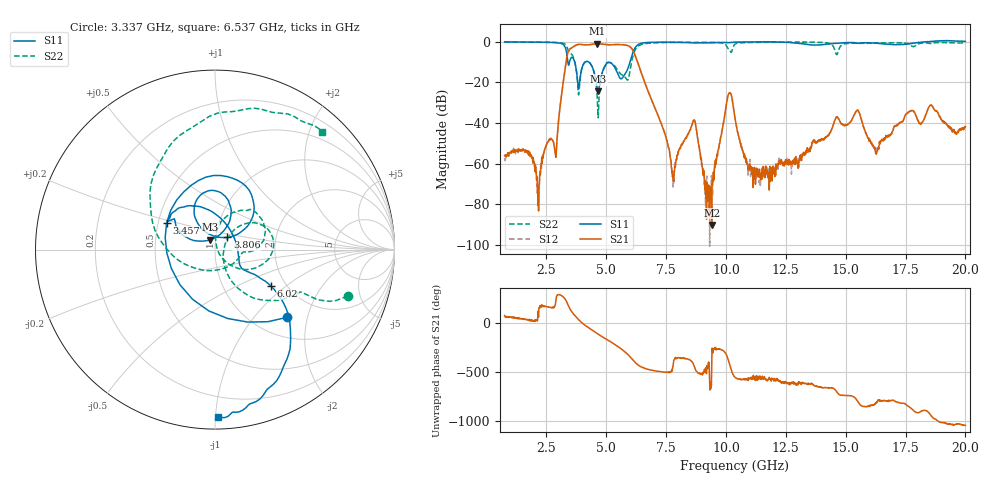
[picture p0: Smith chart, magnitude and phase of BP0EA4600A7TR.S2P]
! s2p File.  Ports: 1,3
# MHz S DB R 50
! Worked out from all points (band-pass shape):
!   1601 points, 750 MHz to 20 GHz, reference 50 ohm
!   highest |S21| = -0.93 dB at 4.624 GHz (marker M1); lowest = -90.3 dB at 9.4 GHz (marker M2)
!   |S21| within 3 dB of the highest: 3.444 GHz to 6.095 GHz (2.651 GHz wide, 55.6 % of centre)
!   lowest |S11| = -24.3 dB at 4.66 GHz (marker M3), VSWR 1.13, Z = 47.2 + j5.22 ohm
!   |S11| at or under -10 dB: 3.393 GHz to 3.462 GHz (68.65 MHz wide, 2 % of centre); 3.677 GHz to 4.111 GHz (433.8 MHz wide, 11.1 % of centre); 4.274 GHz to 5.986 GHz (1.712 GHz wide, 33.4 % of centre)
!   |S22| runs from -37.5 to 0.0 dB; largest |S21 - S12| = 0.0082
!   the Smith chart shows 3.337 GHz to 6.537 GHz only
!   S11 on the Smith chart (normalised r, x): 3.337 GHz: 1.39, -1.51; 3.457 GHz: 0.55, +0.18; 3.806 GHz: 1.14, +0.16; 6.02 GHz: 1.67, -0.79; 6.537 GHz: 0.07, -1.01
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750  0.03 166.4  -56.05 74.5  -57.91 71.9  -0.16 148.6
2169.69  -0.23 119.2  -83.36 59.5  -78.42 -159.4  -0.15 76.1
2903.59  -0.44 70.6  -55.72 -108.9  -55.60 -111.3  -0.32 31.3
3336.72  -5.18 -43.3  -8.41 -142.4  -8.44 -142.6  -2.13 -19.2
3457.03  -10.23 151.2  -3.73 152.1  -3.73 151.9  -5.24 -26.2
3805.94  -20.24 44.4  -1.33 41.2  -1.33 41.1  -21.21 -55.6
3962.34  -13.72 122.1  -1.29 3.7  -1.30 3.6  -13.92 42.7
4624.06  -23.21 86.9  -0.93 -110.2  -0.96 -110.2  -28.58 -46.6
4660.16  -24.31 115.3  -0.95 -116.3  -0.94 -116.4  -37.48 34.1
5550.47  -17.61 44.3  -1.30 106.3  -1.29 106.4  -15.21 -4.1
6019.69  -8.56 -33.1  -2.75 4.5  -2.75 4.6  -12.01 -176.0
6537.03  -0.62 -89.1  -17.87 -99.7  -17.85 -99.7  -1.05 47.7
7174.69  -0.16 -110.0  -36.73 -136.6  -36.83 -136.2  -0.41 -1.0
7800.31  -0.21 -123.0  -67.63 -57.8  -67.94 -46.6  -0.27 -24.0
8678.59  -0.53 -160.5  -38.54 -89.3  -38.45 -90.2  -0.33 -45.2
9400.47  -0.50 156.8  -90.30 -106.6  -67.49 77.3  -0.30 -63.1
10086.25  -0.29 132.1  -26.27 -14.0  -26.32 -13.6  -3.33 -92.4
10375  -0.09 128.7  -37.65 162.6  -37.48 162.2  -1.21 -75.2
11181.09  0.02 125.7  -61.88 148.1  -67.26 171.6  -0.37 -111.0
13587.34  -1.55 59.6  -50.60 100.5  -49.95 100.1  -0.19 -139.7
16799.69  -1.17 -83.5  -46.06 -71.3  -45.66 -79.3  -0.47 127.1
20000  0.17 167.9  -41.74 30.1  -41.96 28.3  -0.55 45.1
